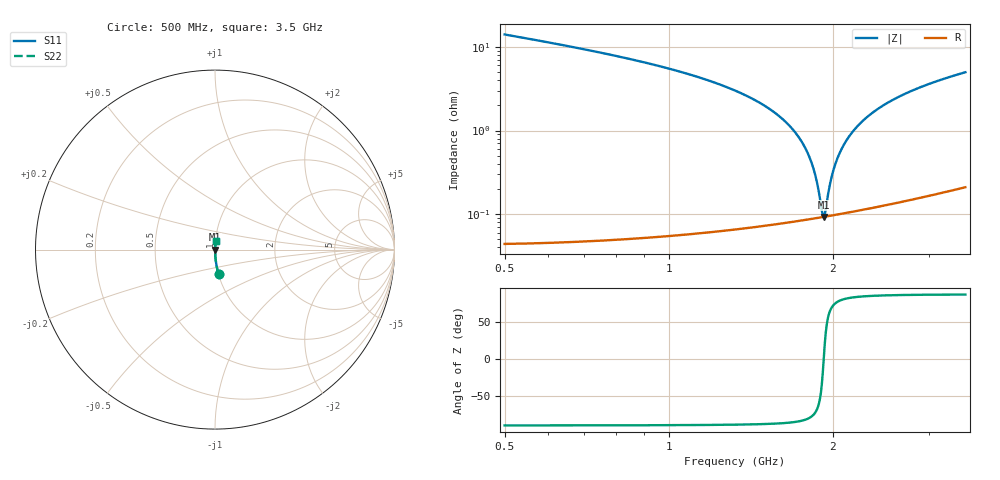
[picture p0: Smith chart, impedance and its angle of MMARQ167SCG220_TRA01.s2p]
! MMARQ167SCG220_TRA01  S-PARAMETER MODEL  ( General Type )
! Model Generated by TAIYO YUDEN Corporation (http://www.ty-top.com)
! Version 1.0
! TAIYO YUDEN Control No. 150305
! Copyright(c) 2015 TAIYO YUDEN CO.,LTD. All Rights Reserved.
! Product Description (link to TY-COMPAS)
! https://ds.yuden.co.jp/TYCOMPAS/or/detail?pn=MMARQ167SCG220JTRA01&u=M
! Products Name : Multilayer Ceramic Capacitors
! Characteristics :
!  Capacitance : 22 pF , Rated Voltage : 250V , TCC : CG / C0G
!  Case Size : 1.6 x 0.8 / 0.063 x 0.031 [mm/inch] , Thickness : 0.7 / 0.028 [mm/inch]
!  (Conditions: Temperature = 25 degC , DC Bias Current/Voltage = 0A / 0V)
! External Node Assignments :
!  1  o---| |---o  2
! GND o---------o GND
! Frequency Range : 500MHz  -  3.5GHz  [ 401 STEP ]
# MHz S RI R 50
! Freq[MHz].  S11 Real  S11 Imag  S21 Real  S21 Imag  S12 Real  S12 Imag  S22 Real  S22 Imag
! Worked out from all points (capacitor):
!   401 points, 500 MHz to 3.5 GHz, reference 50 ohm
!   read as one part in series: C = 21.1 pF near 515 MHz
!   lowest |Z| = 92.8 mohm at 1.925 GHz (marker M1)
!   series resonance near 1.924 GHz, so ESL is about 320 pH
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500  0.0198 -0.1379  0.9802 0.1379  0.9802 0.1379  0.0198 -0.1379
1002.5  0.00354 -0.0546  0.9965 0.0546  0.9965 0.0546  0.00354 -0.0546
1302.5  0.00163 -0.0313  0.9984 0.0313  0.9984 0.0313  0.00163 -0.0313
1505  0.0011 -0.0194  0.9989 0.0194  0.9989 0.0194  0.0011 -0.0194
1662.5  0.000928 -0.0115  0.9991 0.0115  0.9991 0.0115  0.000928 -0.0115
1775  0.00089 -0.00632  0.9991 0.00632  0.9991 0.00632  0.00089 -0.00632
1812.5  0.00089 -0.00468  0.9991 0.00468  0.9991 0.00468  0.00089 -0.00468
1842.5  0.000895 -0.00339  0.9991 0.00339  0.9991 0.00339  0.000895 -0.00339
1872.5  0.000903 -0.00212  0.9991 0.00212  0.9991 0.00212  0.000903 -0.00212
1910  0.000919 -0.000572  0.9991 0.000572  0.9991 0.000572  0.000919 -0.000572
1925  0.000926 4e-05  0.9991 -4e-05  0.9991 -4e-05  0.000926 4e-05
1940  0.000935 0.000648  0.9991 -0.000648  0.9991 -0.000648  0.000935 0.000648
1970  0.000954 0.00185  0.999 -0.00185  0.999 -0.00185  0.000954 0.00185
2000  0.000976 0.00303  0.999 -0.00303  0.999 -0.00303  0.000976 0.00303
2030  0.001 0.0042  0.999 -0.0042  0.999 -0.0042  0.001 0.0042
2067.5  0.00104 0.00563  0.999 -0.00563  0.999 -0.00563  0.00104 0.00563
2172.5  0.00116 0.00953  0.9988 -0.00953  0.9988 -0.00953  0.00116 0.00953
2315  0.00137 0.0146  0.9986 -0.0146  0.9986 -0.0146  0.00137 0.0146
2502.5  0.00171 0.0208  0.9983 -0.0208  0.9983 -0.0208  0.00171 0.0208
2727.5  0.00221 0.0278  0.9978 -0.0278  0.9978 -0.0278  0.00221 0.0278
3005  0.00295 0.0359  0.997 -0.0359  0.997 -0.0359  0.00295 0.0359
3500  0.00454 0.0494  0.9955 -0.0494  0.9955 -0.0494  0.00454 0.0494
